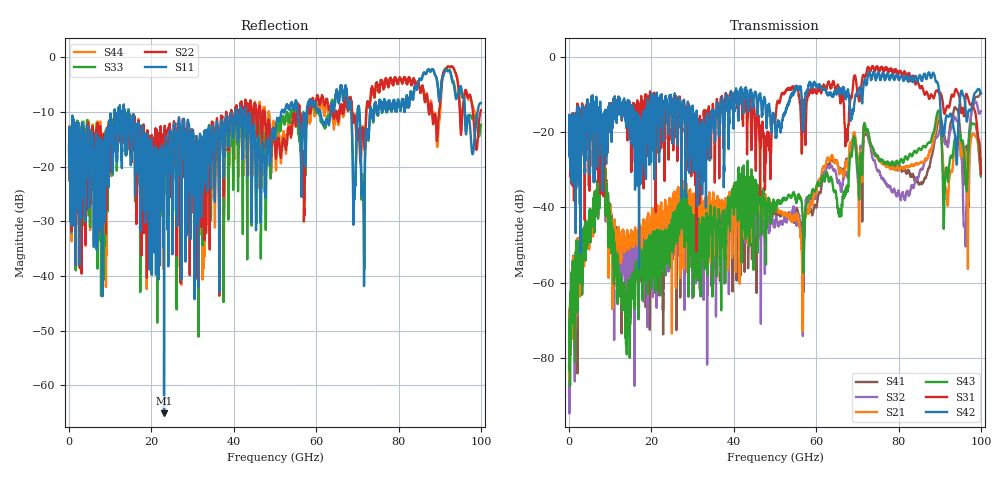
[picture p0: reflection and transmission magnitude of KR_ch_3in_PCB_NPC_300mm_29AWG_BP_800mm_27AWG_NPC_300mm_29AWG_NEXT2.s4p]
# GHz S RI R 45
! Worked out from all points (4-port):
!   4000 points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, 25 MHz to 100 GHz, reference 45 ohm
!   strongest paths, dB at 25 MHz, 25.02 GHz, 50.02 GHz, 75.03 GHz, 100 GHz:
!     S42: -20.6, -18.0, -18.0, -4.3, -9.8
!     S31: -20.6, -13.3, -17.5, -2.9, -31.1
!     S43: -83.1, -45.0, -41.1, -26.4, -31.8
!     S21: -82.3, -46.5, -40.8, -27.2, -27.3
!     S32: -84.5, -44.2, -44.1, -30.5, -14.5
!     S41: -90.4, -50.5, -41.1, -27.1, -9.6
!   lowest |S11| = -65.1 dB at 23.07 GHz (marker M1), VSWR 1.00, Z = 45 + j0.016 ohm
!   |S11| at or under -10 dB: start of sweep to 11.04 GHz; 14.46 GHz to 40.34 GHz (25.88 GHz wide, 94.5 % of centre); 42.82 GHz to 51.62 GHz (8.801 GHz wide, 18.6 % of centre)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
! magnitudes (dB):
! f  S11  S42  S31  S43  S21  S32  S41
! 25 MHz  -16.1  -20.6  -20.6  -83.1  -82.3  -84.5  -90.4
! 8.025 GHz  -17.4  -26.6  -24.1  -24.4  -25.5  -25.3  -24.9
! 13.62 GHz  -12.3  -14.6  -13.8  -67.6  -49.9  -55.1  -55.9
! 23.07 GHz  -65.1  -18.4  -18.7  -47.5  -41.3  -47.4  -45.3
! 93.8 GHz  -7.1  -21.7  -8.8  -21.5  -22.9  -16.1  -13.4
! 96.1 GHz  -9.6  -11.7  -13.2  -28.5  -24.6  -44.6  -27.3
! 100 GHz  -8.4  -9.8  -31.1  -31.8  -27.3  -14.5  -9.6
